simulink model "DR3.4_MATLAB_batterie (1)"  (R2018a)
settings: Solver=VariableStepAuto  StartTime=0.0  StopTime=2  RelTol=1e-3
libraries: fl_lib x5, pe_lib x3, nesl_utility x3

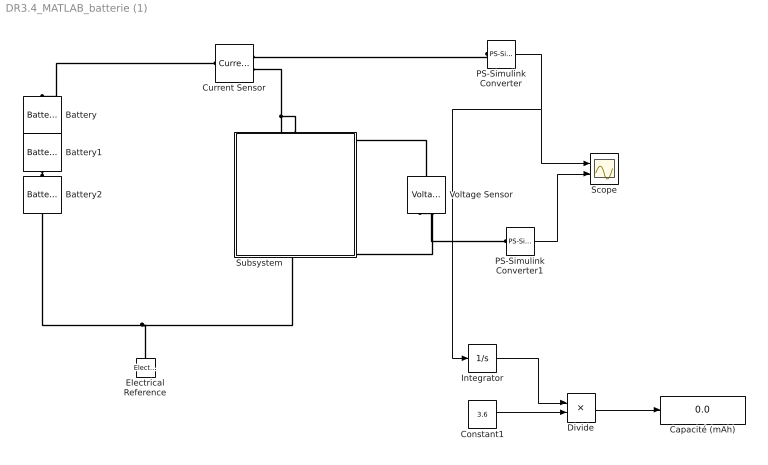
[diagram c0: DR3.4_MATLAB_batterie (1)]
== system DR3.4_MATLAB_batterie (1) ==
  Battery : pe_lib/Sources/Battery  Vnom=1.2 V  R1=0.001 Ohm  prm_AH=2  AH=1.8 hr*A  V1=1 V  AH1=0.4 hr*A  prm_R2=1  R2=2000 Ohm  prm_dyn=1  Rp1=0.005 Ohm  tau1=30 s  Rp2=0.005 Ohm  tau2=30 s  prm_fade=1  N_fade=100  AH_fade=45 hr*A  R1_fade=2.02 Ohm  V1_fade=10.35 V  i_specify=off  i_priority=None  i=0 A  i_nominal_specify=off  i_nominal_unit=A  i_nominal_value=1  v_specify=off  v_priority=None  v=0 V  v_nominal_specify=off  v_nominal_unit=V  v_nominal_value=1  charge_specify=on  charge_priority=High  charge=1.8 hr*A  charge_nominal_specify=off  charge_nominal_unit=hr*A  charge_nominal_value=1  num_cycles_specify=off  num_cycles_priority=High  num_cycles=0  num_cycles_nominal_specify=off  num_cycles_nominal_unit=1  num_cycles_nominal_value=1  thermal_mass=30000 J/K  Tmeas=298.15 K  Vnom_T2=12 V  R1_T2=2.2 Ohm  V1_T2=11.4 V  R2_T2=2200 Ohm  Rp1_T2=0.005 Ohm  tau1_T2=30 s  Rp2_T2=0.005 Ohm  tau2_T2=30 s  Tmeas2=273.15 K  temperature_specify=off  temperature_priority=High  temperature=298.15 K  temperature_nominal_specify=off  temperature_nominal_unit=K  temperature_nominal_value=1
  Battery1 : pe_lib/Sources/Battery  Vnom=1.2 V  R1=0.001 Ohm  prm_AH=2  AH=1.8 hr*A  V1=1 V  AH1=0.4 hr*A  prm_R2=1  R2=2000 Ohm  prm_dyn=1  Rp1=0.005 Ohm  tau1=30 s  Rp2=0.005 Ohm  tau2=30 s  prm_fade=1  N_fade=100  AH_fade=45 hr*A  R1_fade=2.02 Ohm  V1_fade=10.35 V  i_specify=off  i_priority=None  i=0 A  i_nominal_specify=off  i_nominal_unit=A  i_nominal_value=1  v_specify=off  v_priority=None  v=0 V  v_nominal_specify=off  v_nominal_unit=V  v_nominal_value=1  charge_specify=on  charge_priority=High  charge=1.8 hr*A  charge_nominal_specify=off  charge_nominal_unit=hr*A  charge_nominal_value=1  num_cycles_specify=off  num_cycles_priority=High  num_cycles=0  num_cycles_nominal_specify=off  num_cycles_nominal_unit=1  num_cycles_nominal_value=1  thermal_mass=30000 J/K  Tmeas=298.15 K  Vnom_T2=12 V  R1_T2=2.2 Ohm  V1_T2=11.4 V  R2_T2=2200 Ohm  Rp1_T2=0.005 Ohm  tau1_T2=30 s  Rp2_T2=0.005 Ohm  tau2_T2=30 s  Tmeas2=273.15 K  temperature_specify=off  temperature_priority=High  temperature=298.15 K  temperature_nominal_specify=off  temperature_nominal_unit=K  temperature_nominal_value=1
  Battery2 : pe_lib/Sources/Battery  Vnom=1.2 V  R1=0.001 Ohm  prm_AH=2  AH=1.8 hr*A  V1=1 V  AH1=0.4 hr*A  prm_R2=1  R2=2000 Ohm  prm_dyn=1  Rp1=0.005 Ohm  tau1=30 s  Rp2=0.005 Ohm  tau2=30 s  prm_fade=1  N_fade=100  AH_fade=45 hr*A  R1_fade=2.02 Ohm  V1_fade=10.35 V  i_specify=off  i_priority=None  i=0 A  i_nominal_specify=off  i_nominal_unit=A  i_nominal_value=1  v_specify=off  v_priority=None  v=0 V  v_nominal_specify=off  v_nominal_unit=V  v_nominal_value=1  charge_specify=on  charge_priority=High  charge=1.8 hr*A  charge_nominal_specify=off  charge_nominal_unit=hr*A  charge_nominal_value=1  num_cycles_specify=off  num_cycles_priority=High  num_cycles=0  num_cycles_nominal_specify=off  num_cycles_nominal_unit=1  num_cycles_nominal_value=1  thermal_mass=30000 J/K  Tmeas=298.15 K  Vnom_T2=12 V  R1_T2=2.2 Ohm  V1_T2=11.4 V  R2_T2=2200 Ohm  Rp1_T2=0.005 Ohm  tau1_T2=30 s  Rp2_T2=0.005 Ohm  tau2_T2=30 s  Tmeas2=273.15 K  temperature_specify=off  temperature_priority=High  temperature=298.15 K  temperature_nominal_specify=off  temperature_nominal_unit=K  temperature_nominal_value=1
  Capacité (mAh) : Display
  Constant1 : Constant  Value=3.6  VectorParams1D=off
  Current Sensor : fl_lib/Electrical/Electrical Sensors/Current Sensor
  Divide : Product  Inputs=*/
  Electrical Reference : fl_lib/Electrical/Electrical Elements/Electrical Reference
  Integrator : Integrator
  PS-Simulink Converter : nesl_utility/PS-Simulink Converter  PhysicalDomain=network_engine_domain  SubClassName=ps_output  LeftPortType=input  RightPortType=output  PseudoPeriodic=off  Frequencies=[]  Unit=1  AffineConversion=off
  PS-Simulink Converter1 : nesl_utility/PS-Simulink Converter  PhysicalDomain=network_engine_domain  SubClassName=ps_output  LeftPortType=input  RightPortType=output  PseudoPeriodic=off  Frequencies=[]  Unit=1  AffineConversion=off
  Scope : Scope  NumInputPorts=2
  Subsystem : Subsystem  mask{I=1.25}
      mask prompts: I "Intensité consommée (A)"
  Voltage Sensor : fl_lib/Electrical/Electrical Sensors/Voltage Sensor
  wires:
  PS-Simulink Converter/1 -> Integrator/1, Scope/1
  PS-Simulink Converter1/1 -> Scope/2
  Integrator/1 -> Divide/1
  Constant1/1 -> Divide/2
  Divide/1 -> Capacité (mAh)/1
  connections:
  Voltage Sensor/RConn2 -- Subsystem/RConn1 -- Battery2/RConn1 -- Electrical Reference/LConn1
  Current Sensor/LConn1 -- Battery/LConn1
  Current Sensor/RConn2 -- Voltage Sensor/LConn1 -- Subsystem/LConn1
  PS-Simulink Converter/LConn1 -- Current Sensor/RConn1
  PS-Simulink Converter1/LConn1 -- Voltage Sensor/RConn1
  Battery2/LConn1 -- Battery1/RConn1
  Battery/RConn1 -- Battery1/LConn1

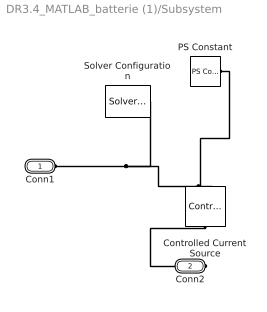
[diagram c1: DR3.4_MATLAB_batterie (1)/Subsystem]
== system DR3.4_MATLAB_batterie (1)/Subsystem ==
  Controlled Current Source : fl_lib/Electrical/Electrical Sources/Controlled Current Source
  PS Constant : fl_lib/Physical Signals/Sources/PS Constant  constant=I
  Solver Configuration : nesl_utility/Solver Configuration  PhysicalDomain=network_engine_domain  SubClassName=solver  LeftPortType=input  RightPortType=generic  Tones=[]  Harmonics=[]  SimulateNoise=off  Profile=off  UseLocalSampling=off  EnableSwitchedLinearOptims=on  FrequencyDomain=off  UseCCode=off  RelTol=0.001  AbsTol=1e-06  MinStep=1e-09  ToWorkspace=off  RevertToSquareIcSolve=off  NumHomotopyIterations=100  PhasorMode=off  PhasorModeNumHarmonics=1  DoDC=off  ResidualTolerance=1e-09  UseLocalSolver=off  LocalSolverChoice=NE_BACKWARD_EULER_ADVANCER  LocalSolverSampleTime=0.001  DoFixedCost=off  MaxNonlinIter=3  MaxModeIter=2  LinearAlgebra=Sparse  EquationFormulation=NE_TIME_EF  DelaysMemoryBudget=1024  AutomaticFiltering=on  FilteringTimeConstant=0.001
  Conn1 : PMIOPort  Side=Left
  Conn2 : PMIOPort  Port=2  Side=Right
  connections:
  Controlled Current Source/LConn1 -- Conn2/RConn1
  Conn1/RConn1 -- Controlled Current Source/RConn2 -- Solver Configuration/RConn1
  PS Constant/RConn1 -- Controlled Current Source/RConn1
